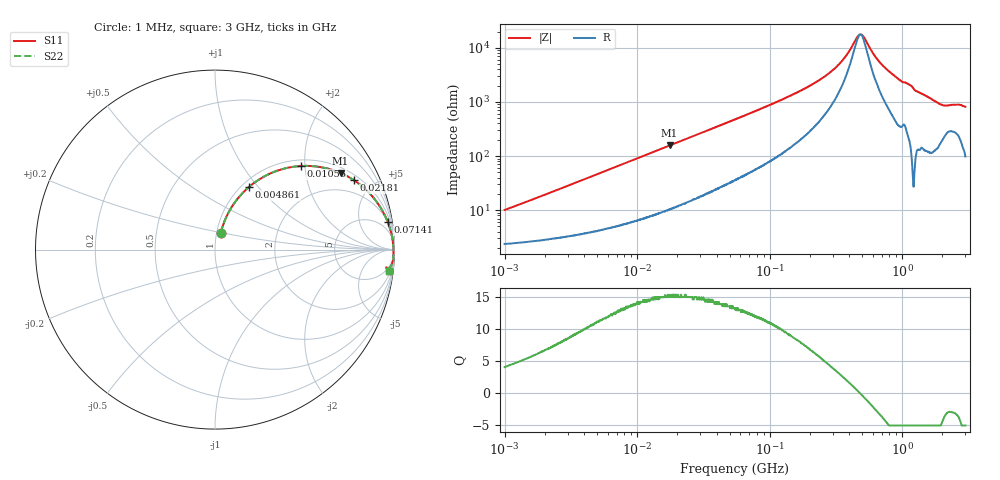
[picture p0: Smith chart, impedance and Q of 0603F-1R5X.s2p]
!s-Parameter Generated by FASTRON Sdn. Bhd.
!FASTRON P/N : 0603F-1R5X
!Keysight Technologies: E4991B_MY54100416_A.01.15
!Date: Wed Jun 19 15:48:55 2024
!Version  :Rev00  Wed Jun 19 15:48:55 2024
!Data & Calibration Information:
!Freq  S11  S21  S12  S22
!PortZ  Port1:50+j0  Port2:50+j0
!When reading reference impedance value at option line is always used.
! Remarks : This data is being provided solely for informational purposes.
# Hz S dB R 50
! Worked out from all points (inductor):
!   1601 points, 1 MHz to 3 GHz, reference 50 ohm
!   read as one part in series: L = 1.54 uH near 1.041 MHz
!   highest Q = 15.1 at 17.59 MHz (marker M1), where L = 1.42 uH
!   self-resonance near 483.7 MHz
!   S11 on the Smith chart (normalised r, x): 1 MHz: 1.05, +0.20; 4.861 MHz: 1.08, +0.90; 10.56 MHz: 1.13, +1.91; 21.81 MHz: 1.26, +3.86; 71.41 MHz: 2, +12; 3 GHz: 3, -16
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1000000  -20.20 70.9  -0.24 -5.5  -0.24 -5.5  -20.20 70.9
2150303  -14.20 70.7  -0.41 -11.2  -0.41 -11.2  -14.20 70.7
3804036  -9.78 65.3  -0.79 -18.8  -0.79 -18.8  -9.78 65.3
4861065  -8.02 61.5  -1.08 -23.3  -1.08 -23.3  -8.02 61.5
1.05579e7  -3.51 44.2  -3.10 -41.7  -3.10 -41.7  -3.51 44.2
1.447069e7  -2.30 36.2  -4.55 -50.0  -4.55 -50.0  -2.30 36.2
1.758912e7  -1.73 31.4  -5.64 -54.8  -5.64 -54.8  -1.73 31.4
2.181181e7  -1.26 26.5  -6.98 -59.7  -6.98 -59.7  -1.26 26.5
3.337442e7  -0.66 18.4  -9.98 -67.6  -9.98 -67.6  -0.66 18.4
5.504702e7  -0.32 11.6  -13.90 -74.1  -13.90 -74.1  -0.32 11.6
7.140691e7  -0.22 9.0  -16.10 -76.4  -16.10 -76.4  -0.22 9.0
2.083556e8  -0.07 2.7  -26.50 -78.7  -26.50 -78.7  -0.07 2.7
3.252521e8  -0.06 1.2  -33.50 -72.0  -33.50 -72.0  -0.06 1.2
3.798301e8  -0.05 0.7  -37.30 -63.4  -37.30 -63.4  -0.05 0.7
4.593788e8  -0.05 0.1  -44.10 -24.5  -44.10 -24.5  -0.05 0.1
4.829509e8  -0.05 0.0  -45.00 -0.8  -45.00 -0.8  -0.05 0.0
5.154121e8  -0.05 -0.2  -43.90 30.0  -43.90 30.0  -0.05 -0.2
6.520712e8  -0.05 -0.9  -35.70 70.1  -35.70 70.1  -0.05 -0.9
7.925923e8  -0.05 -1.5  -31.40 77.1  -31.40 77.1  -0.05 -1.5
1.274982e9  -0.05 -3.6  -24.10 82.6  -24.10 82.6  -0.05 -3.6
1.902655e9  -0.20 -6.0  -19.60 74.3  -19.60 74.3  -0.20 -6.0
3e9  -0.19 -6.9  -18.40 76.2  -18.40 76.2  -0.19 -6.9
